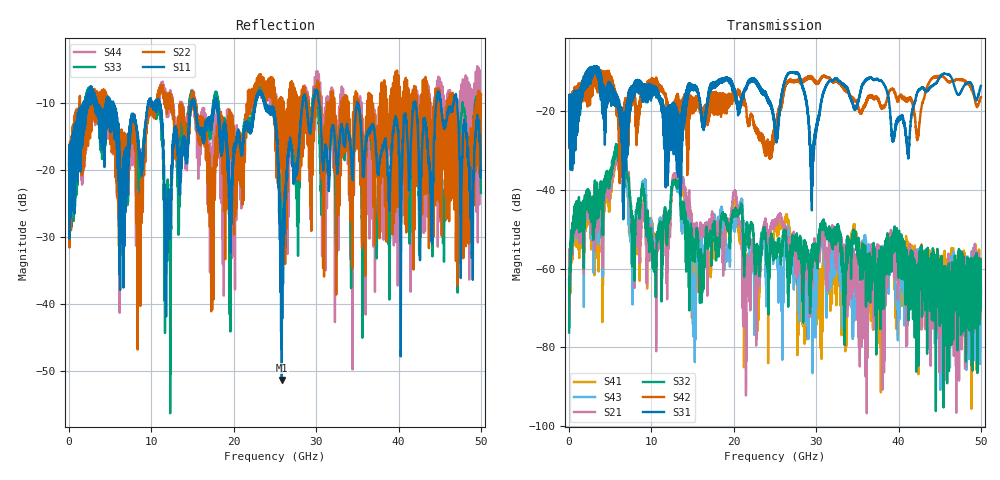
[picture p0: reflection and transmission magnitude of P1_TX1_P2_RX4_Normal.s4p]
!Keysight Technologies,N5225B,MY57041031,A.13.20.10
!Date: Friday, May 31, 2019 11:33:17
!Correction: S11(Full 4 Port(1,2,3,4))
!S12(Full 4 Port(1,2,3,4))
!S13(Full 4 Port(1,2,3,4))
!S14(Full 4 Port(1,2,3,4))
!S21(Full 4 Port(1,2,3,4))
!S22(Full 4 Port(1,2,3,4))
!S23(Full 4 Port(1,2,3,4))
!S24(Full 4 Port(1,2,3,4))
!S31(Full 4 Port(1,2,3,4))
!S32(Full 4 Port(1,2,3,4))
!S33(Full 4 Port(1,2,3,4))
!S34(Full 4 Port(1,2,3,4))
!S41(Full 4 Port(1,2,3,4))
!S42(Full 4 Port(1,2,3,4))
!S43(Full 4 Port(1,2,3,4))
!S44(Full 4 Port(1,2,3,4))
!S4P File: Measurements: <S11,S12,S13,S14>,
!<S21,S22,S23,S24>,
!<S31,S32,S33,S34>,
!<S41,S42,S43,S44>:
# Hz S  dB  R 50.0
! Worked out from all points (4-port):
!   5000 points, 10 MHz to 50 GHz, reference 50 ohm
!   strongest paths, dB at 10 MHz, 12.51 GHz, 25.01 GHz, 37.51 GHz, 50 GHz:
!     S31: -19.4, -29.2, -24.5, -11.8, -13.5
!     S42: -19.6, -27.2, -23.7, -16.9, -16.4
!     S32: -76.2, -38.8, -54.4, -61.1, -64.3
!     S21: -55.1, -39.1, -48.0, -56.2, -66.4
!     S43: -62.7, -39.0, -54.2, -56.9, -64.9
!     S41: -67.5, -39.3, -48.9, -64.7, -65.8
!   lowest |S11| = -51.3 dB at 25.83 GHz (marker M1), VSWR 1.01, Z = 49.9 + j0.265 ohm
!   |S11| at or under -10 dB: 17.97 GHz to 22.61 GHz (4.636 GHz wide, 22.9 % of centre); 30.38 GHz to 34.95 GHz (4.564 GHz wide, 14 % of centre); 34.98 GHz to 41.82 GHz (6.843 GHz wide, 17.8 % of centre)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
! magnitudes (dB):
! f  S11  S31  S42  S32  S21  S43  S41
! 10 MHz  -19.9  -19.4  -19.6  -76.2  -55.1  -62.7  -67.5
! 5.71 GHz  -15.1  -17.9  -16.9  -28.3  -30.0  -29.2  -30.9
! 15.16 GHz  -9.7  -14.0  -16.5  -56.0  -50.2  -63.5  -59.0
! 20.13 GHz  -17.0  -15.2  -17.0  -46.4  -40.0  -50.4  -42.3
! 21.33 GHz  -13.9  -14.6  -17.9  -55.0  -69.5  -57.5  -62.8
! 25.83 GHz  -51.3  -16.0  -18.4  -54.4  -48.0  -64.9  -48.8
! 50 GHz  -19.7  -13.5  -16.4  -64.3  -66.4  -64.9  -65.8
